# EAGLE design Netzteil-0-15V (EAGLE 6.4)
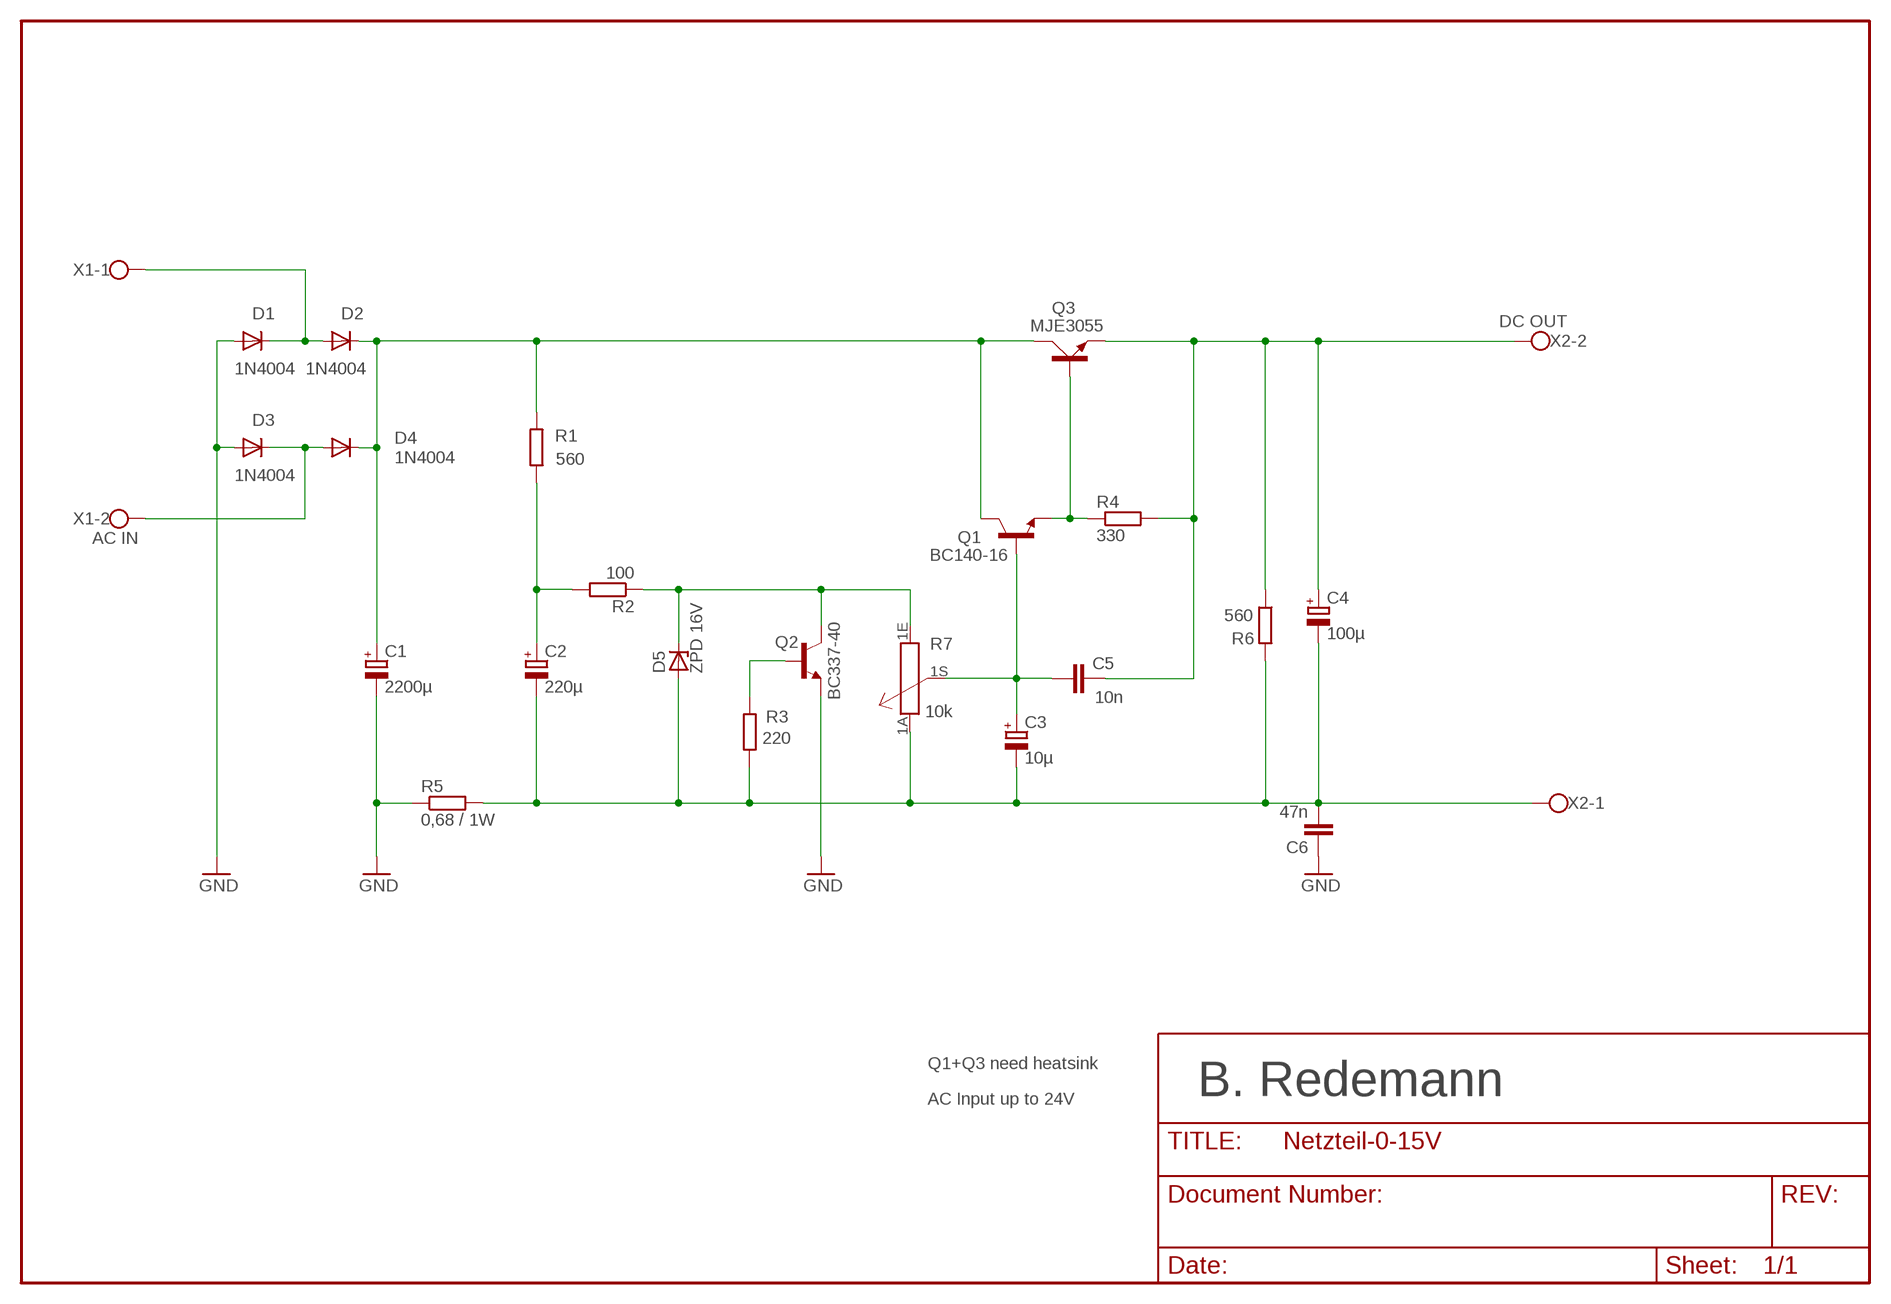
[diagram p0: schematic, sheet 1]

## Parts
C1  2200µ  CPOL-EUE35-12AXIAL  [E35-12]
C2  220µ  CPOL-EUE2.5-7  [E2,5-7]
C3  10µ  CPOL-EUE1.8-4  [E1,8-4]
C4  100µ  CPOL-EUE2.5-7  [E2,5-7]
C5  10n  C-EU025-024X044  [C025-024X044]
C6  47n  C-EU025-024X044  [C025-024X044]
D1  1N4004  [DO41-10]
D2  1N4004  [DO41-10]
D3  1N4004  [DO41-10]
D4  1N4004  [DO41-10]
D5  ZPD 16V  ZPD  [DO35Z10]
Q1  BC140-16  [TO39]
Q2  BC337-40  [TO92]
Q3  MJE3055  [TO220AV]
R1  560  R-EU_0207/10  [0207/10]
R2  100  R-EU_0207/10  [0207/10]
R3  220  R-EU_0207/10  [0207/10]
R4  330  R-EU_0207/10  [0207/10]
R5  0,68 / 1W  R-EU_RDH/15  [RDH/15]
R6  560  R-EU_0207/10  [0207/10]
R7  10k  PC16S  [PC16S]
X1  AC IN  W237-02P  [W237-132]
X2  DC OUT  W237-02P  [W237-132]

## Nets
GND: C1.- C6.1 D1.A D3.A Q2.1(E) R5.1
GND-OUT: C2.- C3.- C4.- C6.2 D5.A R3.2 R5.2 R6.2 R7.1A X2.1
N$1: Q2.2(B) R3.1
N$2: C2.+ R1.1 R2.2
N$3: D5.C Q2.3(C) R2.1 R7.1E
N$5: C1.+ D2.C D4.C Q1.3(C) Q3.C R1.2
N$6: C3.+ C5.1 Q1.2(B) R7.1S
N$7: D1.C D2.A X1.1
N$8: D3.C D4.A X1.2
N$9: Q1.1(E) Q3.B R4.1
N$10: C4.+ C5.2 Q3.E R4.2 R6.1 X2.2

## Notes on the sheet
- Q1+Q3 need heatsink
- B. Redemann
- AC Input up to 24V

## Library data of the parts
C1-C4 = rcl:CPOL-EU: POLARIZED CAPACITOR, European symbol
C5 C6 = rcl:C-EU: CAPACITOR, European symbol
D1-D4 = diode:1N4004: DIODE
D5 = diode:ZPD: Z DIODE
Q1 = transistor-npn:BC140-16: NPN Transistor
Q2 = transistor-npn:BC337*: NPN Transistor
Q3 = transistor-power:MJE3055: NPN TRANSISTOR
R1-R6 = rcl:R-EU_: RESISTOR, European symbol
R7 = piher:PC16S: POTENTIOMETER single carbon potentiometer, 16 mm, S3ROH
X1 X2 = con-wago-508:W237-02P: WAGO SREW CLAMP

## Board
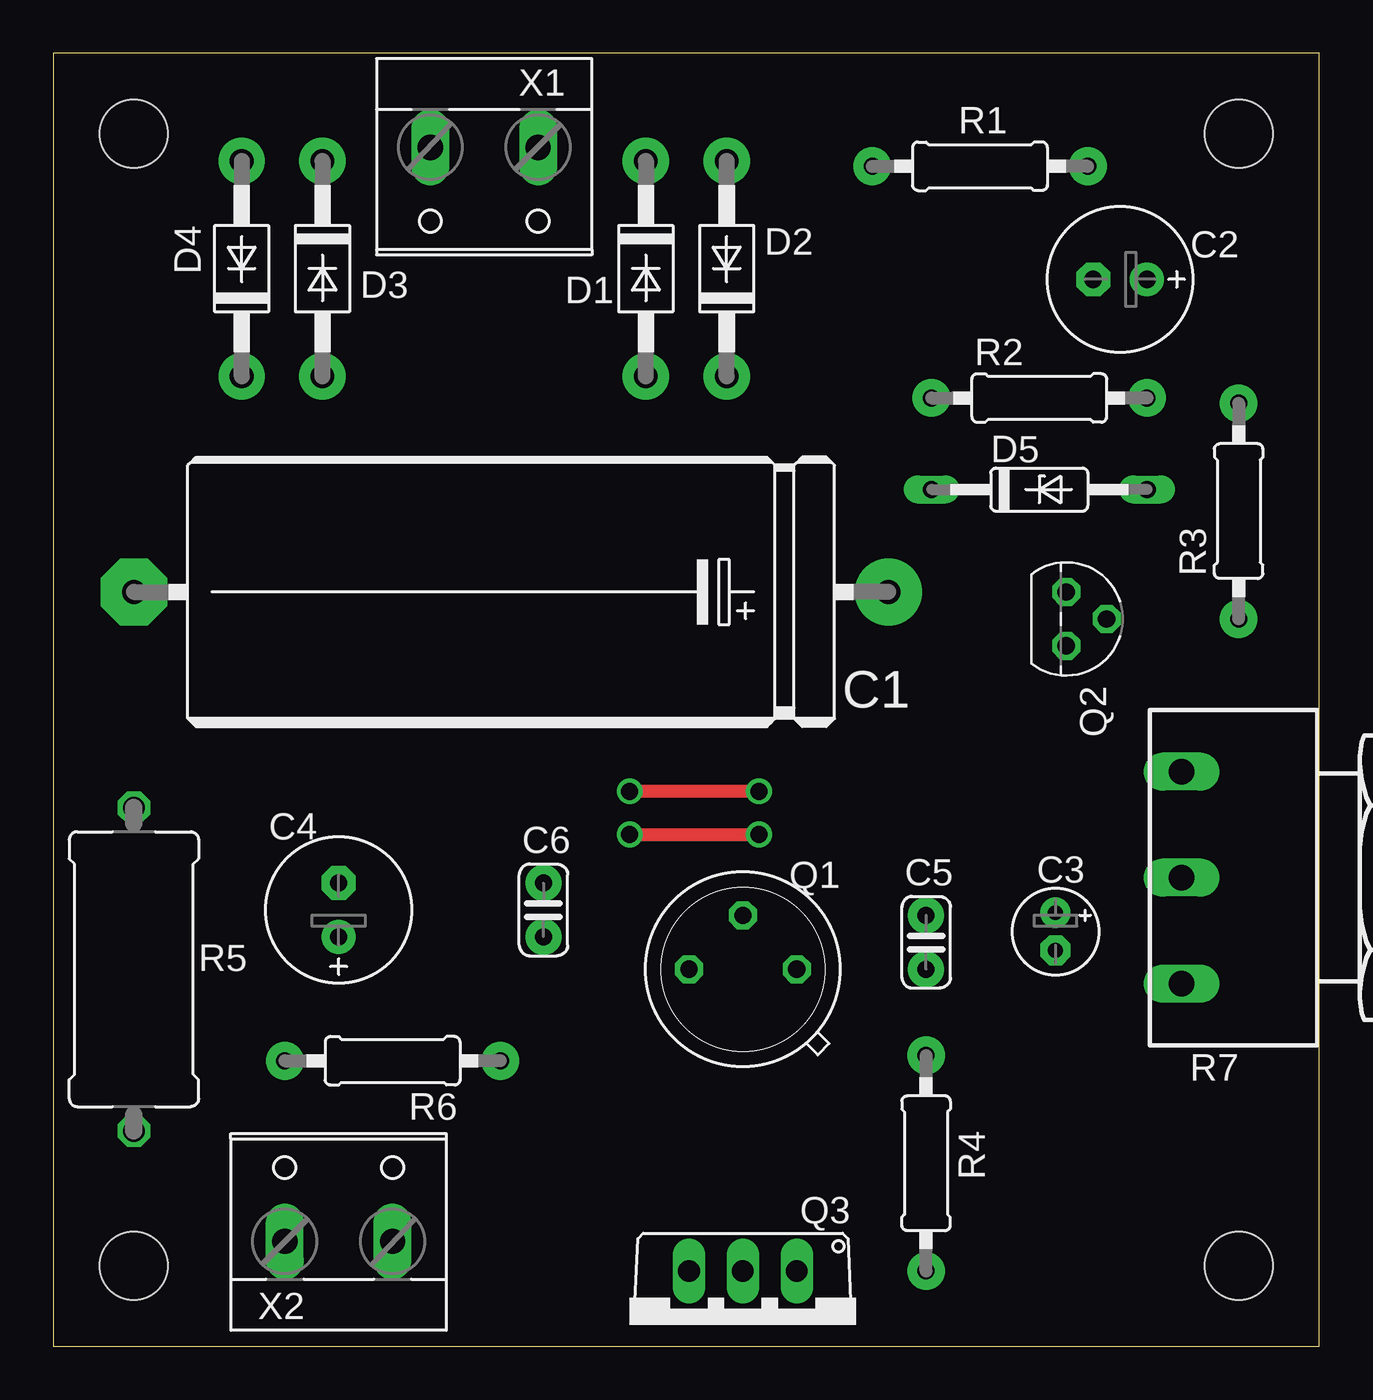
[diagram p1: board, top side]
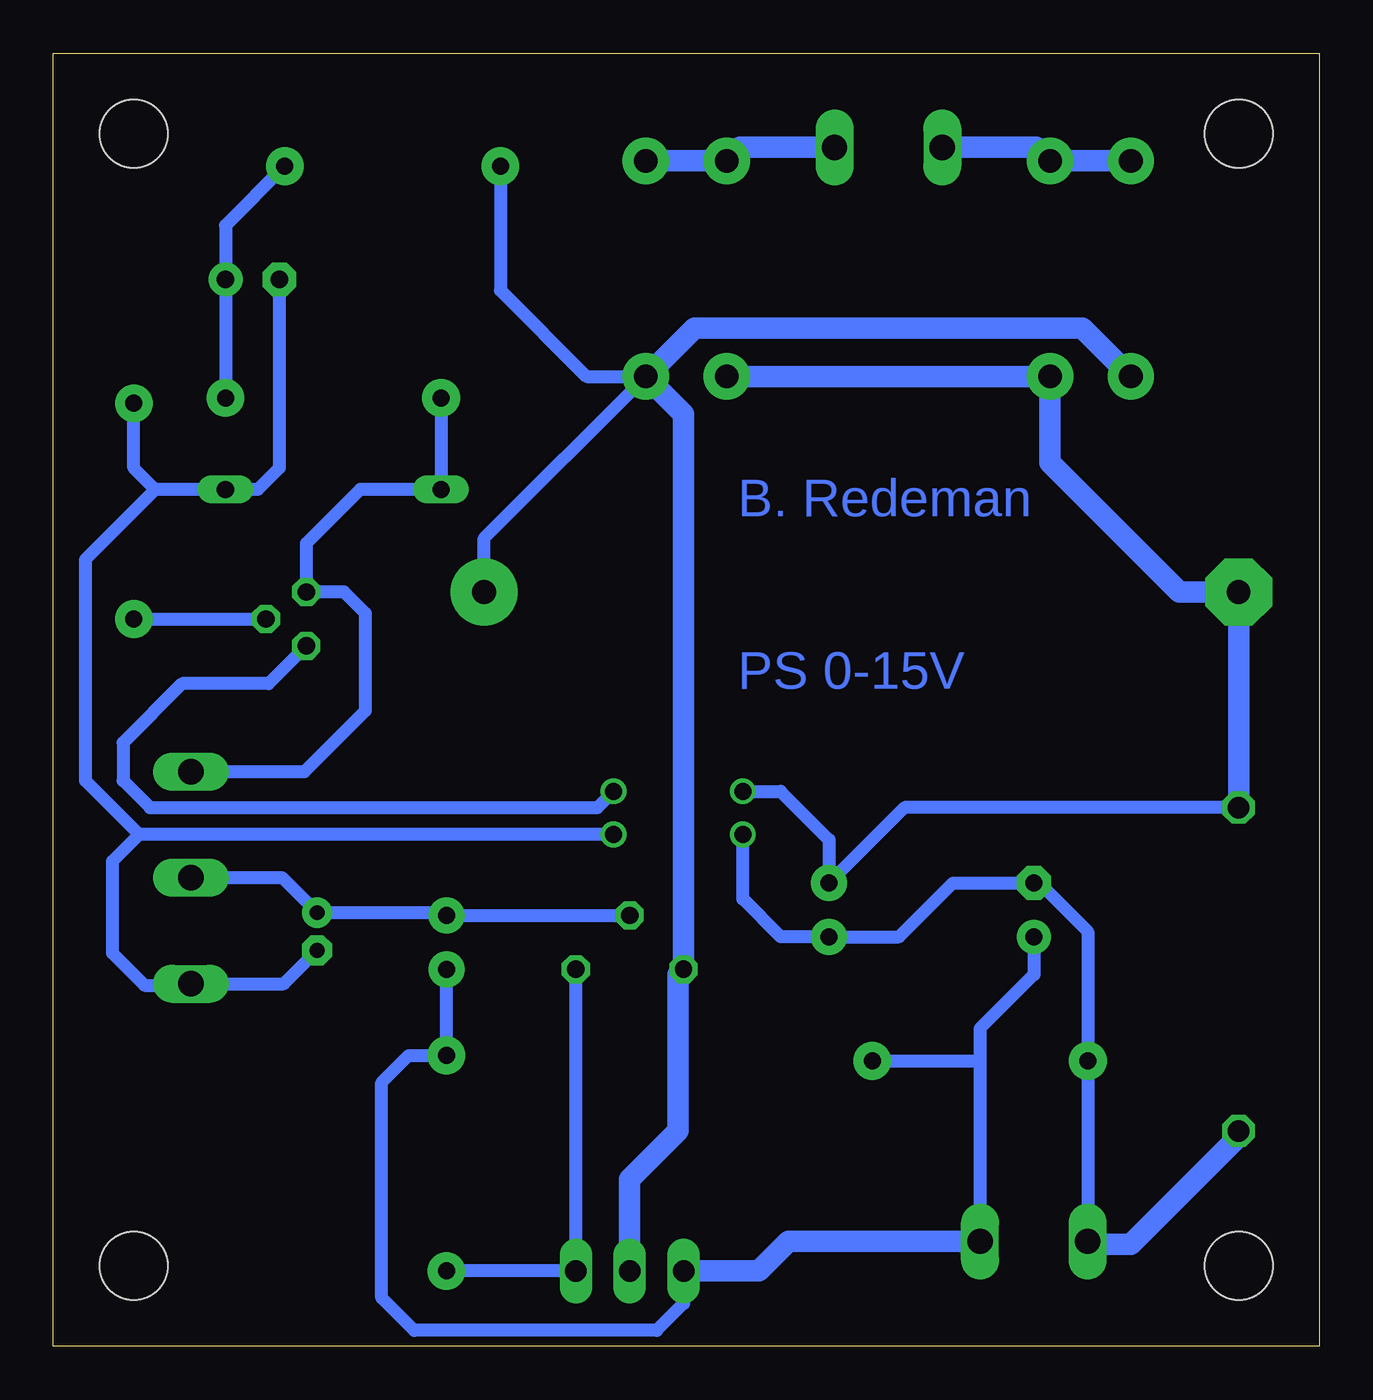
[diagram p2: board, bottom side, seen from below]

Size 59.69 x 60.96 mm. Coordinates in mm from the lower left corner, seen from the top.
Outline: 0,0 59.69,0 59.69,60.96 0,60.96 0,0
Copper layers (1*16): Top 0.035mm / dielectric 1.5mm / Bottom 0.035mm
Design rules "default": minimum track width 10mil, minimum drill 24mil, track to track 8mil, track to pad 8mil, pad to pad 8mil, via to via 8mil, smd to smd 8mil, copper to edge 40mil, drill to drill 8mil, minimum pad ring 10mil, minimum via ring 8mil, stop-mask expansion 4mil, vias tented up to drill 0mil, thermal gap 10mil
Holes 3.2 mm at 3.81,57.15 55.88,57.15 55.88,3.81 3.81,3.81

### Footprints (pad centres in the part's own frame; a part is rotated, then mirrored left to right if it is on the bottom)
E35-12 = drill 1.118 pad 3.15: + -17.78,0 | drill 1.118 pad 3.15 octagon: - 17.78,0
E2,5-7 = drill 0.813 pad 1.6: + -1.27,0 | drill 0.813 pad 1.6 octagon: - 1.27,0
E1,8-4 = drill 0.7 pad 1.422: + -0.889,0 | drill 0.7 pad 1.422 octagon: - 0.889,0
C025-024X044 = drill 0.8 pad 1.7: 1 -1.27,0; 2 1.27,0
DO41-10 = drill 1.118 pad 2.184: A 5.08,0; C -5.08,0
DO35Z10 = drill 0.813 long: A 5.08,0; C -5.08,0
TO39 = drill 0.813 octagon: 1 0,-2.54; 2 2.54,0; 3 0,2.54
TO92 = drill 0.813 octagon: 1 1.27,0; 2 0,1.905; 3 -1.27,0
TO220AV = drill 1.016 long: B -2.54,-2.54; C 0,-2.54; E 2.54,-2.54
0207/10 = drill 0.8 pad 1.778: 1 -5.08,0; 2 5.08,0
RDH/15 = drill 1.016 octagon: 1 -7.62,0; 2 7.62,0
PC16S = drill 1.2 long: 1A -5,6.5; 1E 5,6.5; 1S 0,6.5
W237-132 = drill 1.194 long: 1 -2.54,-0.635; 2 2.54,-0.635

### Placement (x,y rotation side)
C1  21.59,35.56 180 top
C2  50.29,50.29 180 top
C3  47.24,19.56 270 top
C4  13.46,20.57 90 top
C5  41.15,19.05 270 top
C6  23.11,20.57 270 top
D1  27.94,50.8 270 top
D2  31.75,50.8 90 top
D3  12.7,50.8 270 top
D4  8.89,50.8 90 top
D5  46.48,40.39 0 top
Q1  32.51,17.78 90 top
Q2  47.75,34.29 270 top
Q3  32.51,1.02 180 top
R1  43.69,55.63 180 top
R2  46.48,44.7 0 top
R3  55.88,39.37 90 top
R4  41.15,8.64 90 top
R5  3.81,17.78 270 top
R6  16,13.46 180 top
R7  59.69,22.1 90 top
X1  20.32,55.88 180 top
X2  13.46,5.59 0 top

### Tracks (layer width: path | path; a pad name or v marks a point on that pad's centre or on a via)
GND  (via drill 0.8)
  Top 0.61: v33.27,26.16 v27.18,26.16
  Bottom 0.61: R5.1 19.56,25.4 C6.1 23.11,23.88 25.4,26.16 v27.18,26.16 | Q2.1 49.53,31.24 53.59,31.24 56.39,28.45 56.39,26.67 55.12,25.4 34.04,25.4 v33.27,26.16
  Bottom 1.016: D1.A D3.A 12.7,41.66 6.6,35.56 C1.- R5.1
GND-OUT  (via drill 0.8)
  Top 0.61: v27.18,24.13 v33.27,24.13
  Bottom 0.61: C2.- 49.02,41.4 50.04,40.39 D5.A 54.86,40.39 | 54.86,40.39 55.88,41.4 R3.2 | X2.1 R6.2 10.92,19.56 13.21,21.84 C4.- 17.27,21.84 19.81,19.3 C6.2 25.4,19.3 27.18,21.08 v27.18,24.13 | C3.- 48.81,17.1 R7.1A 53.27,17.02 55.37,17.02 56.9,18.54 56.9,22.86 55.63,24.13 | 54.86,40.39 58.17,37.08 58.17,26.67 55.63,24.13 | v33.27,24.13 55.63,24.13
  Bottom 1.016: R5.2 3.81,9.91 8.89,4.83 10.79,4.83 X2.1
N$1
  Bottom 0.61: R3.1 Q2.2
N$2
  Bottom 0.61: R1.1 51.56,52.83 C2.+ R2.2
N$3
  Bottom 0.61: R2.1 D5.C 45.21,40.39 47.75,37.85 Q2.3 45.97,35.56 44.96,34.54 44.96,29.97 47.83,27.1 R7.1E
N$5
  Bottom 0.61: R1.2 38.61,49.78 34.54,45.72 D2.C 39.37,38.1 C1.+
  Bottom 1.016: D4.C 11.18,48.01 29.46,48.01 D2.C 29.97,43.94 Q1.3 30.23,17.53 30.23,10.16 32.51,7.87 Q3.C
N$6
  Bottom 0.61: R7.1S 48.9,22.1 C3.+ 41.27,20.45 C5.1 Q1.2
N$7
  Bottom 1.016: X1.1 27.3,56.52 D1.C D2.A
N$8
  Bottom 1.016: X1.2 13.34,56.52 D3.C D4.A
N$9
  Bottom 0.61: Q1.1 Q3.B R4.1
N$10
  Bottom 0.61: C4.+ 13.46,17.53 16,14.99 16,13.46 | 16,13.46 X2.2 | R6.1 16,13.46 | C5.2 R4.2 42.93,13.72 44.2,12.45 44.2,2.29 42.67,0.76 31.24,0.76 29.97,2.03 Q3.E
  Bottom 1.016: X2.2 25.02,4.95 26.42,3.56 Q3.E

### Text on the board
Bottom: B. Redeman | PS 0-15V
